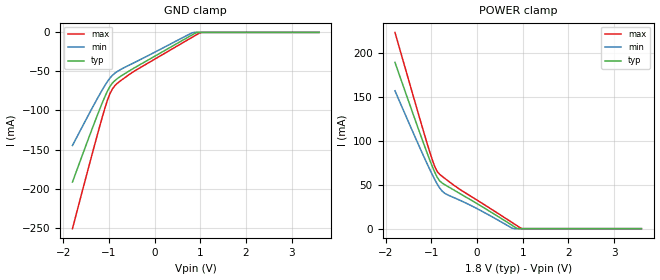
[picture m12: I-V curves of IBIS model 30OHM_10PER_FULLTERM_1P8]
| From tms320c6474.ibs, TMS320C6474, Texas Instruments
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|   Model Cell 30OHM_10PER_FULLTERM_1P8
|30OHM_10PER_FULLTERM_1P8
[Model]   30OHM_10PER_FULLTERM_1P8
Model_type   Input
Polarity   Non-Inverting
Vinl =  0.8
Vinh =  1
C_comp   1.89p   1.72p   2.18p
[Model Spec]
Vinl   0.8   0.71   0.89
Vinh   1   0.91   1.09
D_overshoot_high 2.34 NA NA
D_overshoot_low -0.54 NA NA
D_overshoot_time 0.56n NA NA
S_overshoot_high 2.2 NA NA
S_overshoot_low -0.4 NA NA
[Receiver Thresholds]
Vth = 0.9V
Vth_min = 0.855V
Vth_max = 0.945V
Vinl_dc = -125mV
Vinh_dc = +125mV
Vinl_ac = -250mV
Vinh_ac = +250mV
Tslew_ac = 5.000ns
Threshold_sensitivity = 0.50
Reference_supply Pullup_ref
[Temperature Range]   25   125   -40
[Voltage Range]   1.8   1.62   1.98
[Pullup reference]   1.8   1.62   1.98
[POWER_clamp]
|   voltage   I(typ)   I(min)   I(max)
-1.8V     189.6mA    157.3mA    223.8mA
-1.2V     101.1mA    85.89mA    115.5mA
-981.8mV  70.89mA    61.53mA    78.43mA
-927.3mV  64.18mA    55.91mA    70.65mA
-872.7mV  58.44mA    50.7mA     64.98mA
-763.6mV  51.95mA    42.68mA    59.55mA
-654.5mV  48.52mA    38.75mA    55.22mA
-381.8mV  40.13mA    32.48mA    44.92mA
763.6mV   3.898mA    598.3uA    7.094mA
872.7mV   299.8uA    0A         3.409mA
981.8mV   0A         0A         0A
3.6V      0A         0A         0A
[GND_clamp]
|   voltage   I(typ)   I(min)   I(max)
-1.8V     -191.7mA   -144.8mA   -251.4mA
-1.364V   -122.7mA   -96.4mA    -154.7mA
-1.091V   -82.44mA   -68.14mA   -97.31mA
-1.036V   -75.46mA   -63.18mA   -87.18mA
-981.8mV  -69.5mA    -58.75mA   -78.7mA
-927.3mV  -65.05mA   -55.11mA   -72.69mA
-818.2mV  -59.22mA   -50.09mA   -65.21mA
-436.4mV  -45.18mA   -38.42mA   -49.32mA
818.2mV   -3.311mA   -553.9uA   -6.4mA
927.3mV   0A         0A         -2.692mA
1.036V    0A         0A         0A
3.6V      0A         0A         0A
